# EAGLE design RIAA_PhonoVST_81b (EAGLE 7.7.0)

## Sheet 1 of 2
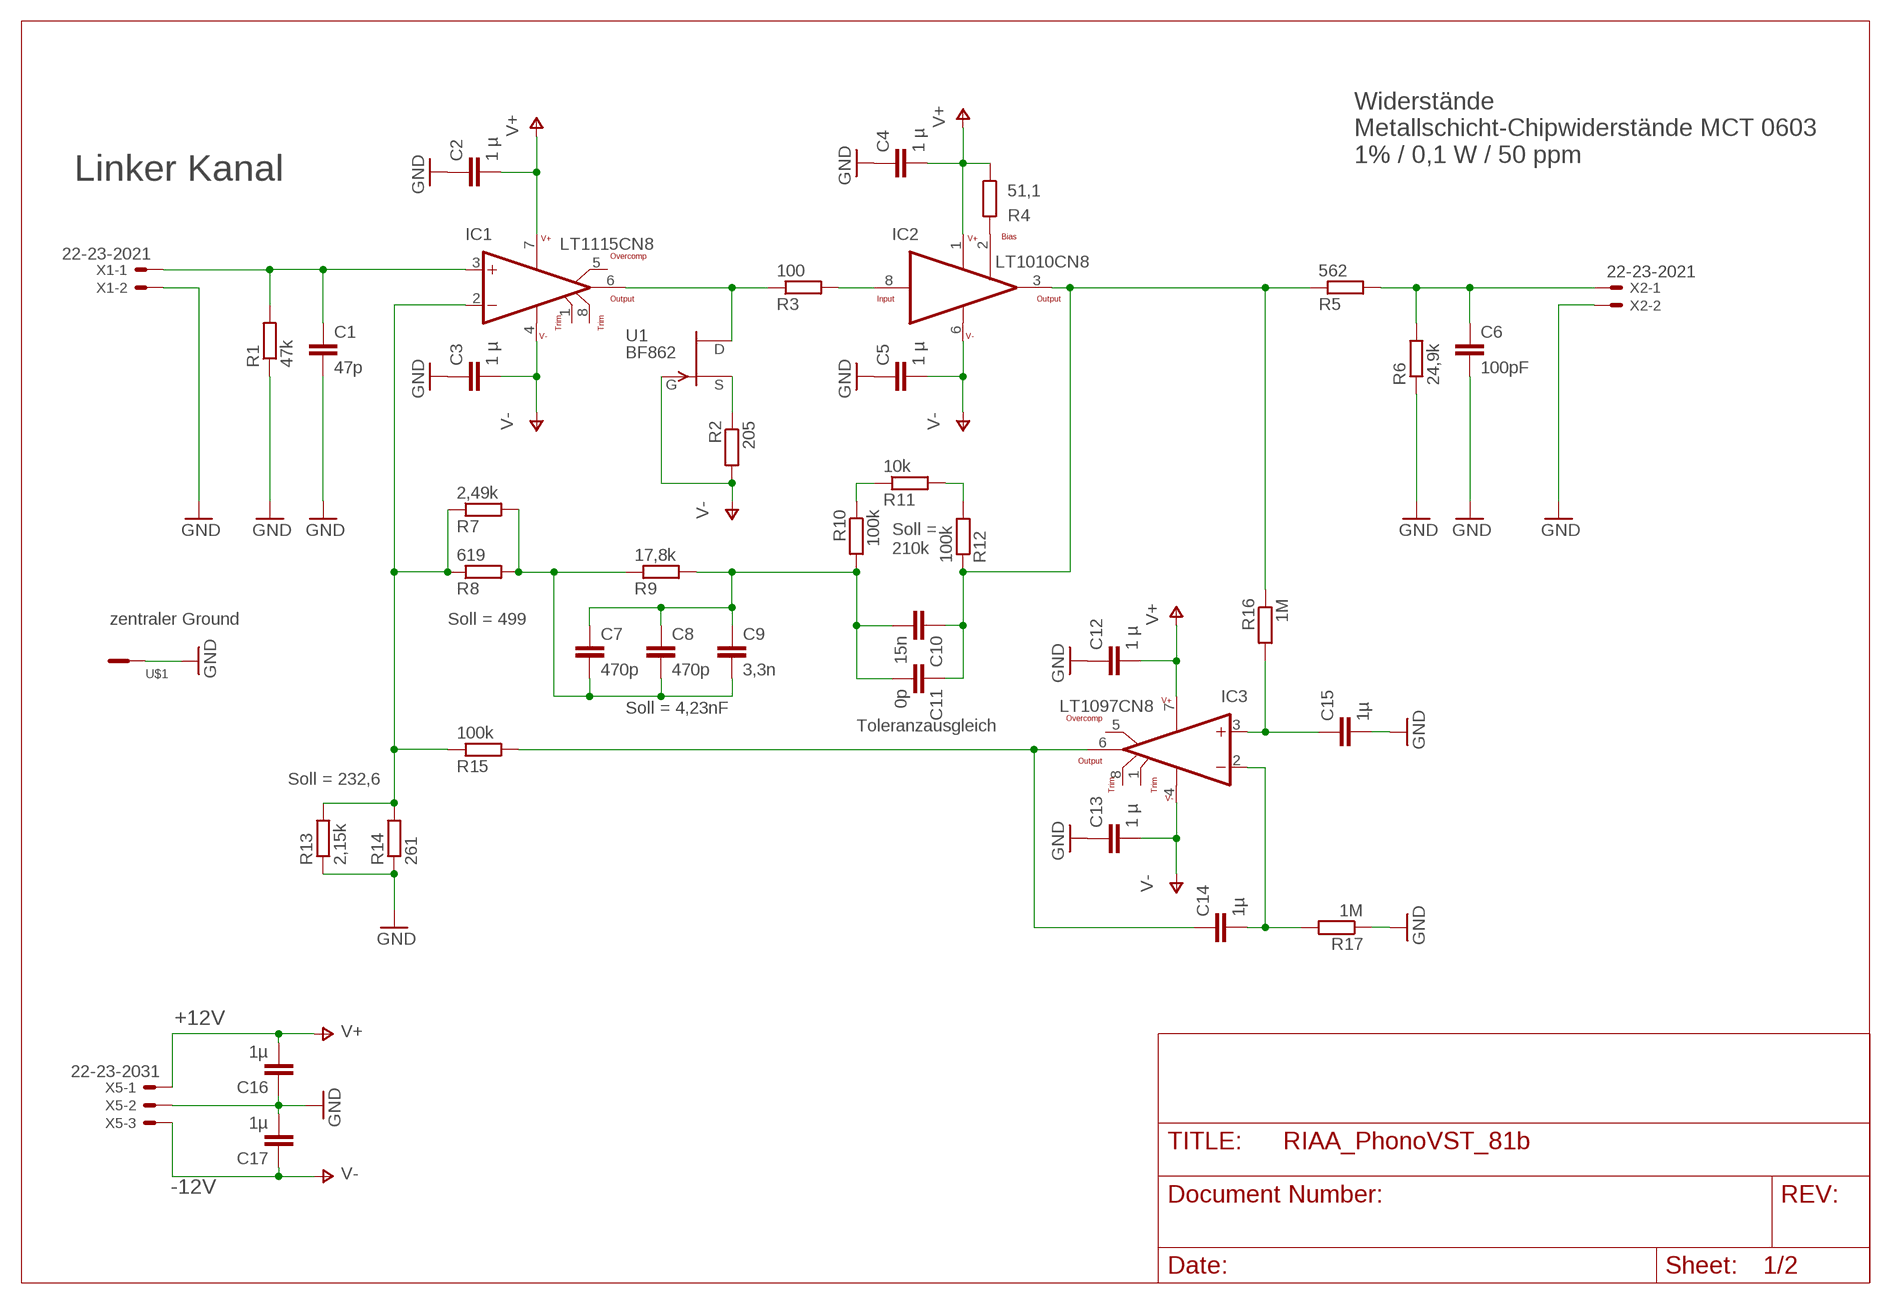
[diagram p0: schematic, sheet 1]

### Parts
C1  47p  C-EUC0603  [C0603]
C2  1 µ  C-EUC1206  [C1206]
C3  1 µ  C-EUC1206  [C1206]
C4  1 µ  C-EUC1206  [C1206]
C5  1 µ  C-EUC1206  [C1206]
C6  100pF  C-EUC0805  [C0805]
C7  470p  C-EUC2012  [C2012]
C8  470p  C-EUC2012  [C2012]
C9  3,3n  C-EUC3225  [C3225]
C10  15n  C-EUC3225  [C3225]
C11  0p  C-EUC2012  [C2012]
C12  1 µ  C-EUC1206  [C1206]
C13  1 µ  C-EUC1206  [C1206]
C14  1µ  C-EUC1206  [C1206]
C15  1µ  C-EUC1206  [C1206]
C16  1µ  C-EUC1206  [C1206]
C17  1µ  C-EUC1206  [C1206]
IC1  LT1115CN8  [DIL08]
IC2  LT1010CN8  [DIL08]
IC3  LT1097CN8  [DIL08]
R1  47k  R-EU_R0603  [R0603]
R2  205  R-EU_R0603  [R0603]
R3  100  R-EU_R0603  [R0603]
R4  51,1  R-EU_R0603  [R0603]
R5  562  R-EU_R0603  [R0603]
R6  24,9k  R-EU_R0603  [R0603]
R7  2,49k  R-EU_R0603  [R0603]
R8  619  R-EU_R0603  [R0603]
R9  17,8k  R-EU_R0603  [R0603]
R10  100k  R-EU_R0603  [R0603]
R11  10k  R-EU_R0603  [R0603]
R12  100k  R-EU_R0603  [R0603]
R13  2,15k  R-EU_R0603  [R0603]
R14  261  R-EU_R0603  [R0603]
R15  100k  R-EU_R0603  [R0603]
R16  1M  R-EU_R0603  [R0603]
R17  1M  R-EU_R0603  [R0603]
U1  BF862  [SOT23]
U$1  2FEET  [2FEETS]
X1  22-23-2021  [22-23-2021]
X2  22-23-2021  [22-23-2021]
X5  22-23-2031  [22-23-2031]

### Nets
GND: C1.2 C2.1 C3.1 C4.1 C5.1 C6.2 C12.1 C13.1 C15.2 C16.1 C17.2 R1.1 R6.1 R13.1 R14.1 R17.1 U$1.P$1 X1.2 X2.2 X5.2 ; also sheet 2
IC1: C1.1 IC1.3(+IN) R1.2 X1.1
IC2: IC2.8(INPUT) R3.2
IC3: C15.1 IC3.3(+IN) R16.2
N$1: C14.1 IC3.6(OUTPUT) R15.2
N$2: R2.1 U1.1(S)
N$3: IC2.2(BIAS) R4.2
N$5: C6.1 R5.2 R6.2 X2.1
N$7: C7.2 C8.2 C9.2 R7.2 R8.2 R9.1
N$8: C7.1 C8.1 C9.1 C10.2 C11.2 R9.2 R10.2
N$9: C14.2 IC3.2(-IN) R17.2
N$10: IC1.6(OUTPUT) R3.1 U1.2(D)
N$11: C10.1 C11.1 IC2.3(OUTPUT) R5.1 R12.1 R16.1
N$12: IC1.2(-IN) R7.1 R8.1 R13.2 R14.2 R15.1
N$13: R10.1 R11.1
N$17: R11.2 R12.2
V+: C2.2 C4.2 C12.2 C16.2 IC1.7(V+) IC2.1(V+) IC3.7(V+) R4.1 X5.1 ; also sheet 2
V-: C3.2 C5.2 C13.2 C17.1 IC1.4(V-) IC2.6(V-) IC3.4(V-) R2.2 U1.3(G) X5.3 ; also sheet 2
Unconnected: IC1.1(TRIM1) IC1.5(OVERCOMP) IC1.8(TRIM2) IC3.1(TRIM1) IC3.5(OVERCOMP) IC3.8(TRIM2)

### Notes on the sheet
- Widerstände
  Metallschicht-Chipwiderstände MCT 0603
  1% / 0,1 W / 50 ppm
- Linker Kanal
- Soll =
  210k
- zentraler Ground | Soll = 499
- Soll = 4,23nF
- Toleranzausgleich
- Soll = 232,6
- +12V
- -12V

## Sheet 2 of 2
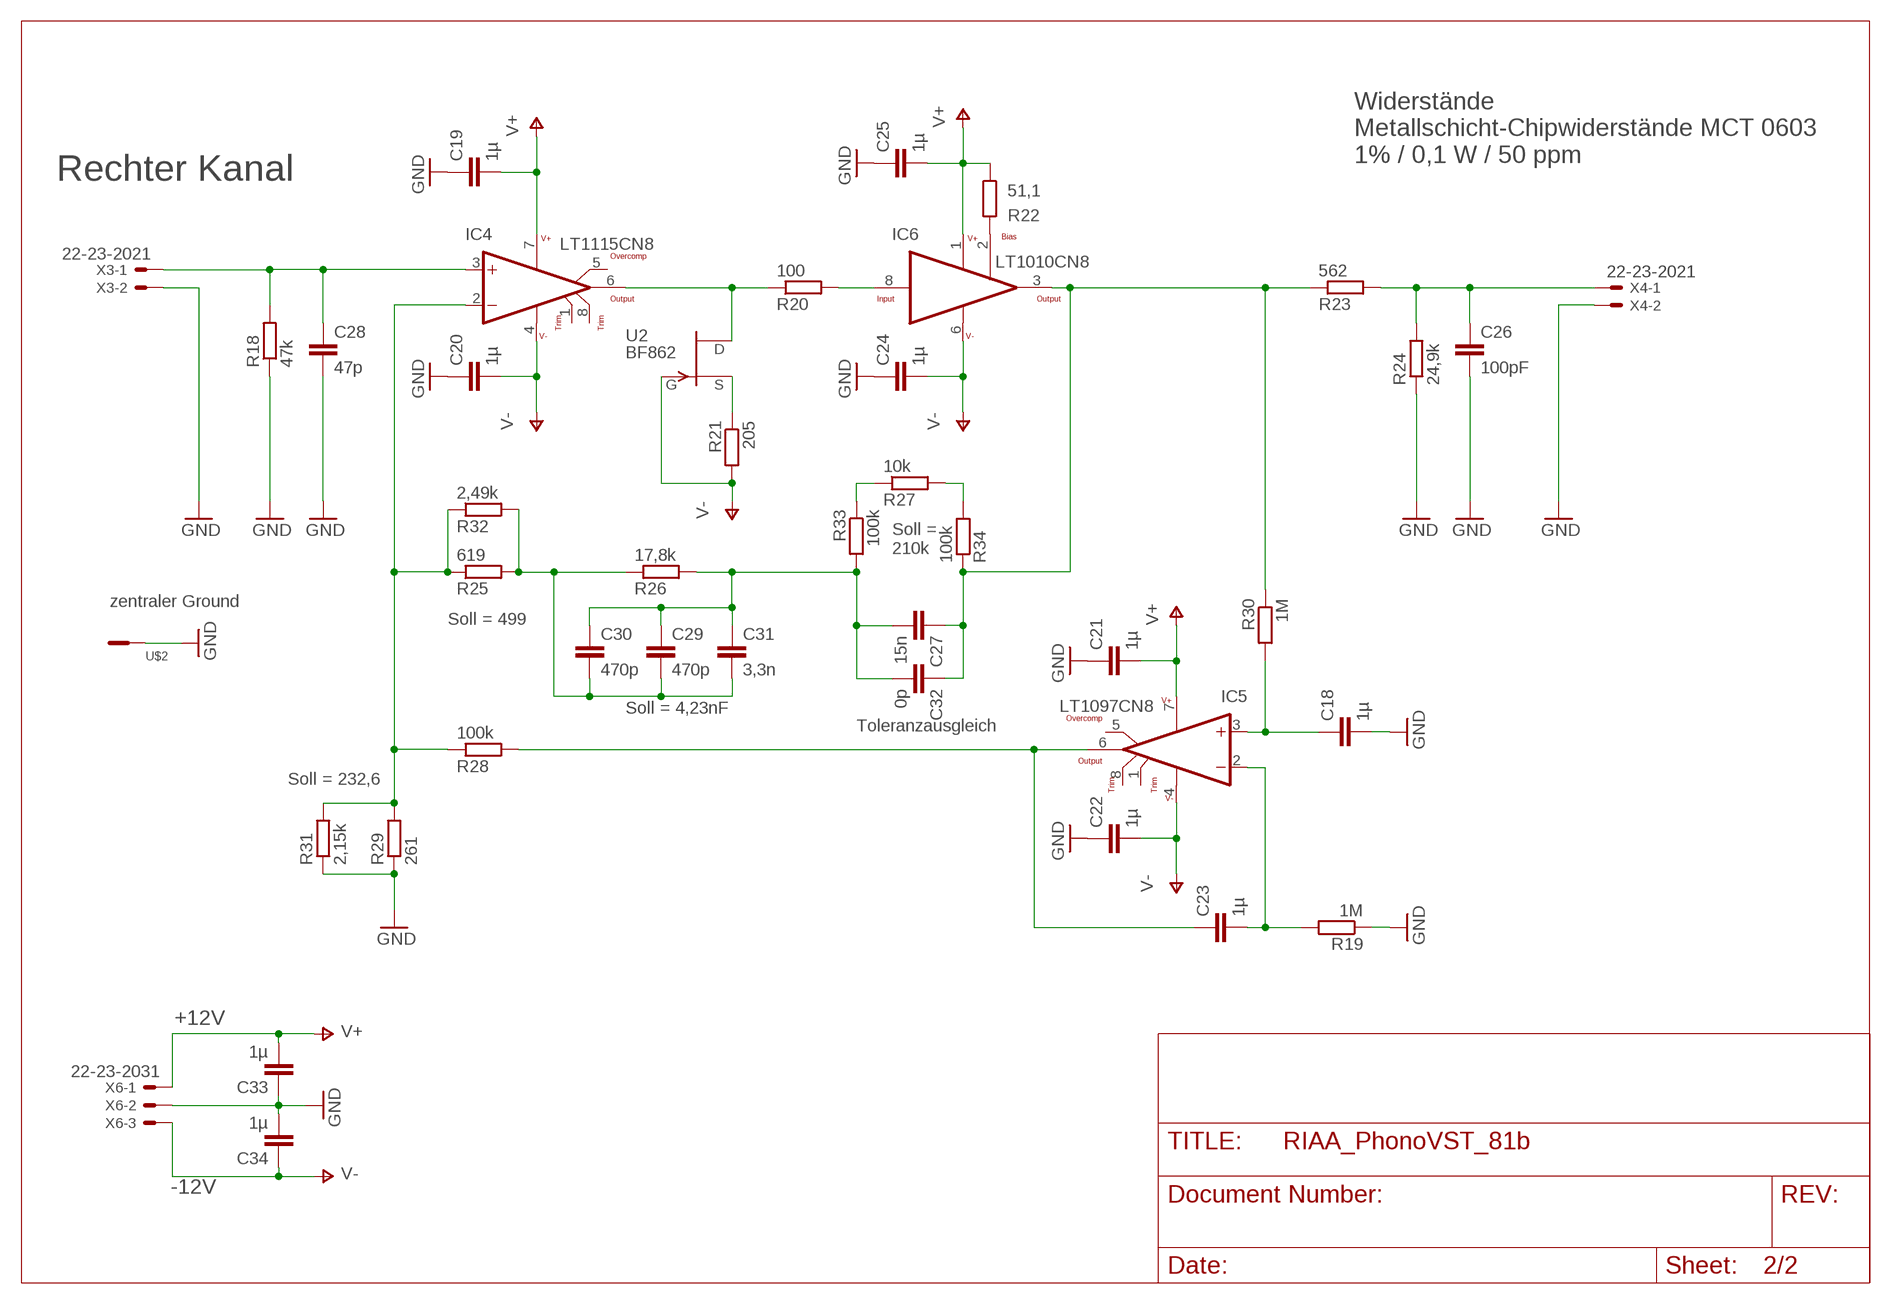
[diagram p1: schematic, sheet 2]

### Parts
C18  1µ  C-EUC1206  [C1206]
C19  1µ  C-EUC1206  [C1206]
C20  1µ  C-EUC1206  [C1206]
C21  1µ  C-EUC1206  [C1206]
C22  1µ  C-EUC1206  [C1206]
C23  1µ  C-EUC1206  [C1206]
C24  1µ  C-EUC1206  [C1206]
C25  1µ  C-EUC1206  [C1206]
C26  100pF  C-EUC0805  [C0805]
C27  15n  C-EUC3225  [C3225]
C28  47p  C-EUC0603  [C0603]
C29  470p  C-EUC2012  [C2012]
C30  470p  C-EUC2012  [C2012]
C31  3,3n  C-EUC3225  [C3225]
C32  0p  C-EUC2012  [C2012]
C33  1µ  C-EUC1206  [C1206]
C34  1µ  C-EUC1206  [C1206]
IC4  LT1115CN8  [DIL08]
IC5  LT1097CN8  [DIL08]
IC6  LT1010CN8  [DIL08]
R18  47k  R-EU_R0603  [R0603]
R19  1M  R-EU_R0603  [R0603]
R20  100  R-EU_R0603  [R0603]
R21  205  R-EU_R0603  [R0603]
R22  51,1  R-EU_R0603  [R0603]
R23  562  R-EU_R0603  [R0603]
R24  24,9k  R-EU_R0603  [R0603]
R25  619  R-EU_R0603  [R0603]
R26  17,8k  R-EU_R0603  [R0603]
R27  10k  R-EU_R0603  [R0603]
R28  100k  R-EU_R0603  [R0603]
R29  261  R-EU_R0603  [R0603]
R30  1M  R-EU_R0603  [R0603]
R31  2,15k  R-EU_R0603  [R0603]
R32  2,49k  R-EU_R0603  [R0603]
R33  100k  R-EU_R0603  [R0603]
R34  100k  R-EU_R0603  [R0603]
U2  BF862  [SOT23]
U$2  2FEET  [2FEETS]
X3  22-23-2021  [22-23-2021]
X4  22-23-2021  [22-23-2021]
X6  22-23-2031  [22-23-2031]

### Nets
GND: C18.2 C19.1 C20.1 C21.1 C22.1 C24.1 C25.1 C26.2 C28.2 C33.1 C34.2 R18.1 R19.1 R24.1 R29.1 R31.1 U$2.P$1 X3.2 X4.2 X6.2 ; also sheet 1
IC4: C28.1 IC4.3(+IN) R18.2 X3.1
IC5: IC6.8(INPUT) R20.2
IC6: C18.1 IC5.3(+IN) R30.2
N$18: C23.2 IC5.2(-IN) R19.2
N$19: IC4.6(OUTPUT) R20.1 U2.2(D)
N$20: C27.1 C32.1 IC6.3(OUTPUT) R23.1 R30.1 R34.1
N$21: C23.1 IC5.6(OUTPUT) R28.2
N$22: R21.1 U2.1(S)
N$23: IC6.2(BIAS) R22.2
N$24: C26.1 R23.2 R24.2 X4.1
N$25: C29.2 C30.2 C31.2 R25.2 R26.1 R32.2
N$26: C27.2 C29.1 C30.1 C31.1 C32.2 R26.2 R33.2
N$27: IC4.2(-IN) R25.1 R28.1 R29.2 R31.2 R32.1
N$28: R27.1 R33.1
N$29: R27.2 R34.2
V+: C19.2 C21.2 C25.2 C33.2 IC4.7(V+) IC5.7(V+) IC6.1(V+) R22.1 X6.1 ; also sheet 1
V-: C20.2 C22.2 C24.2 C34.1 IC4.4(V-) IC5.4(V-) IC6.6(V-) R21.2 U2.3(G) X6.3 ; also sheet 1
Unconnected: IC4.1(TRIM1) IC4.5(OVERCOMP) IC4.8(TRIM2) IC5.1(TRIM1) IC5.5(OVERCOMP) IC5.8(TRIM2)

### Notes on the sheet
- Widerstände
  Metallschicht-Chipwiderstände MCT 0603
  1% / 0,1 W / 50 ppm
- Rechter Kanal
- Soll =
  210k
- zentraler Ground
- Soll = 499
- Soll = 4,23nF
- Toleranzausgleich
- Soll = 232,6
- +12V
- -12V

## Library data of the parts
C1-C34 = rcl:C-EU: CAPACITOR, European symbol
IC1 IC4 = linear-technology:LT1115: Ultra-Low Noise, Low Distortion, Audio Op Amp
IC2 IC6 = linear-technology:LT1010: Fast ±150mA Power Buffer, Very Low Distortion Operation, 20MHz Bandwidth
IC3 IC5 = linear-technology:LT1097: Low Cost, Low Power Precision Op Amp
R1-R34 = rcl:R-EU_: RESISTOR, European symbol
U1 U2 = transistor-fet:BF862: N-channel junction FET
U$1 U$2 = Steckzungen:2FEET: Steckzunge Steckbreite: 2.8 mm Steckdicke: 0.8 mm 180 ° Unisoliert Metall Vogt Verbindungstechnik 3785q08.68
X1-X4 = con-molex:22-23-2021: .100" (2.54mm) Center Header - 2 Pin; MF: MOLEX; MPN: 22-23-2021; OC_FARNELL: 1462926; OC_NEWARK: 25C3832
X5 X6 = con-molex:22-23-2031: .100" (2.54mm) Center Header - 3 Pin; MF: MOLEX; MPN: 22-23-2031; OC_FARNELL: 1462950; OC_NEWARK: 30C0862

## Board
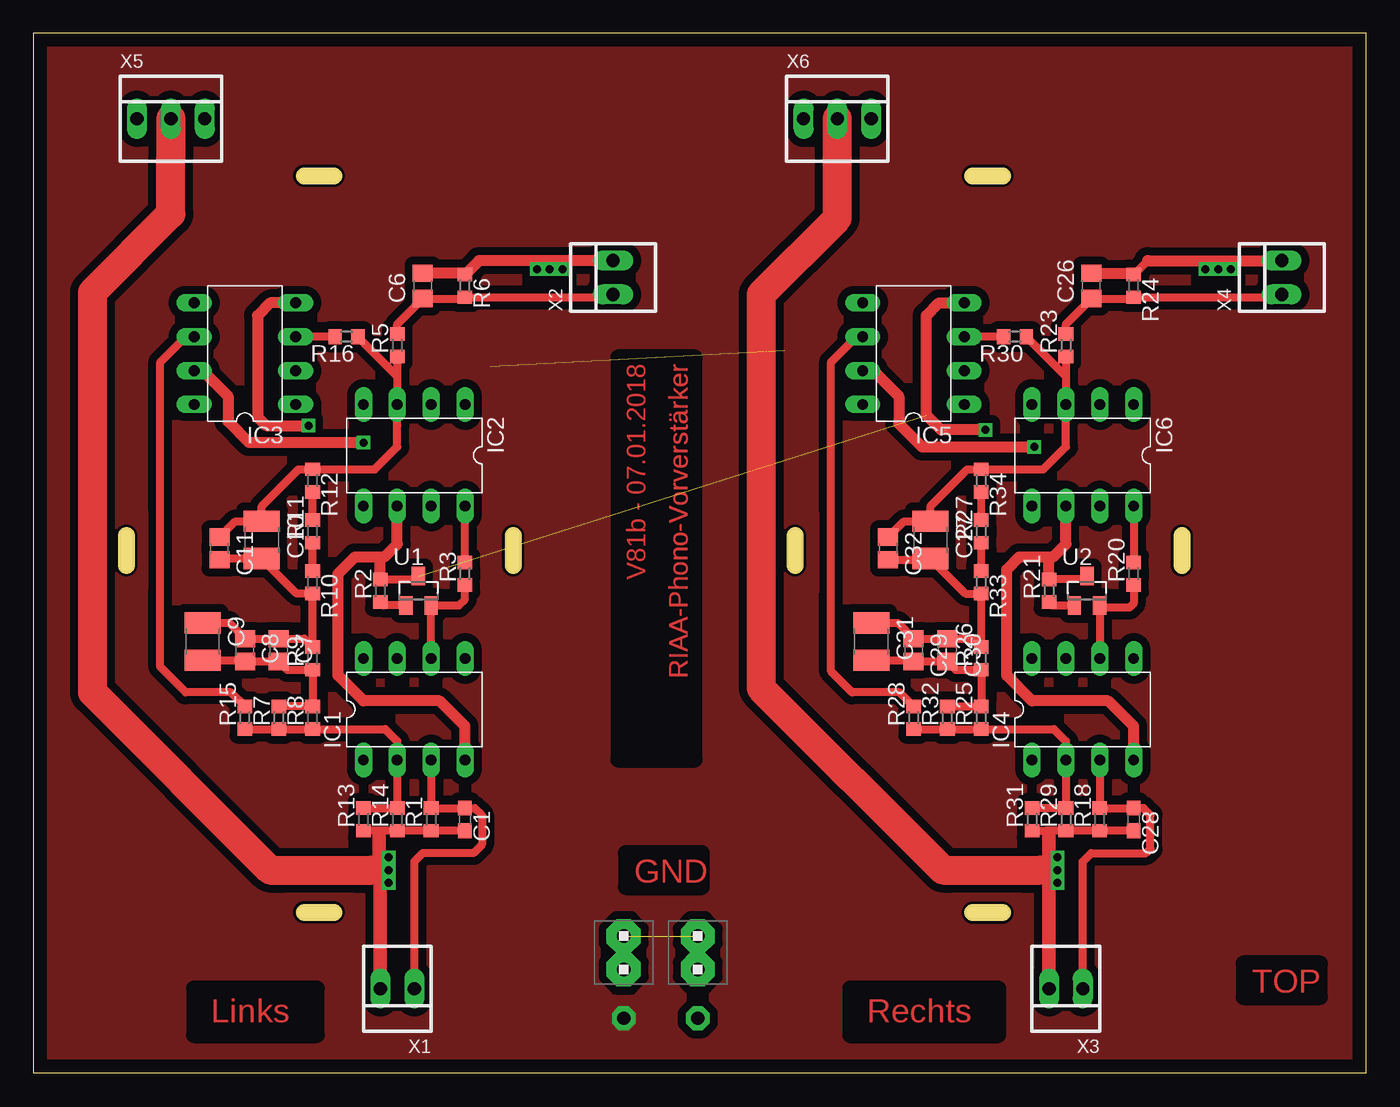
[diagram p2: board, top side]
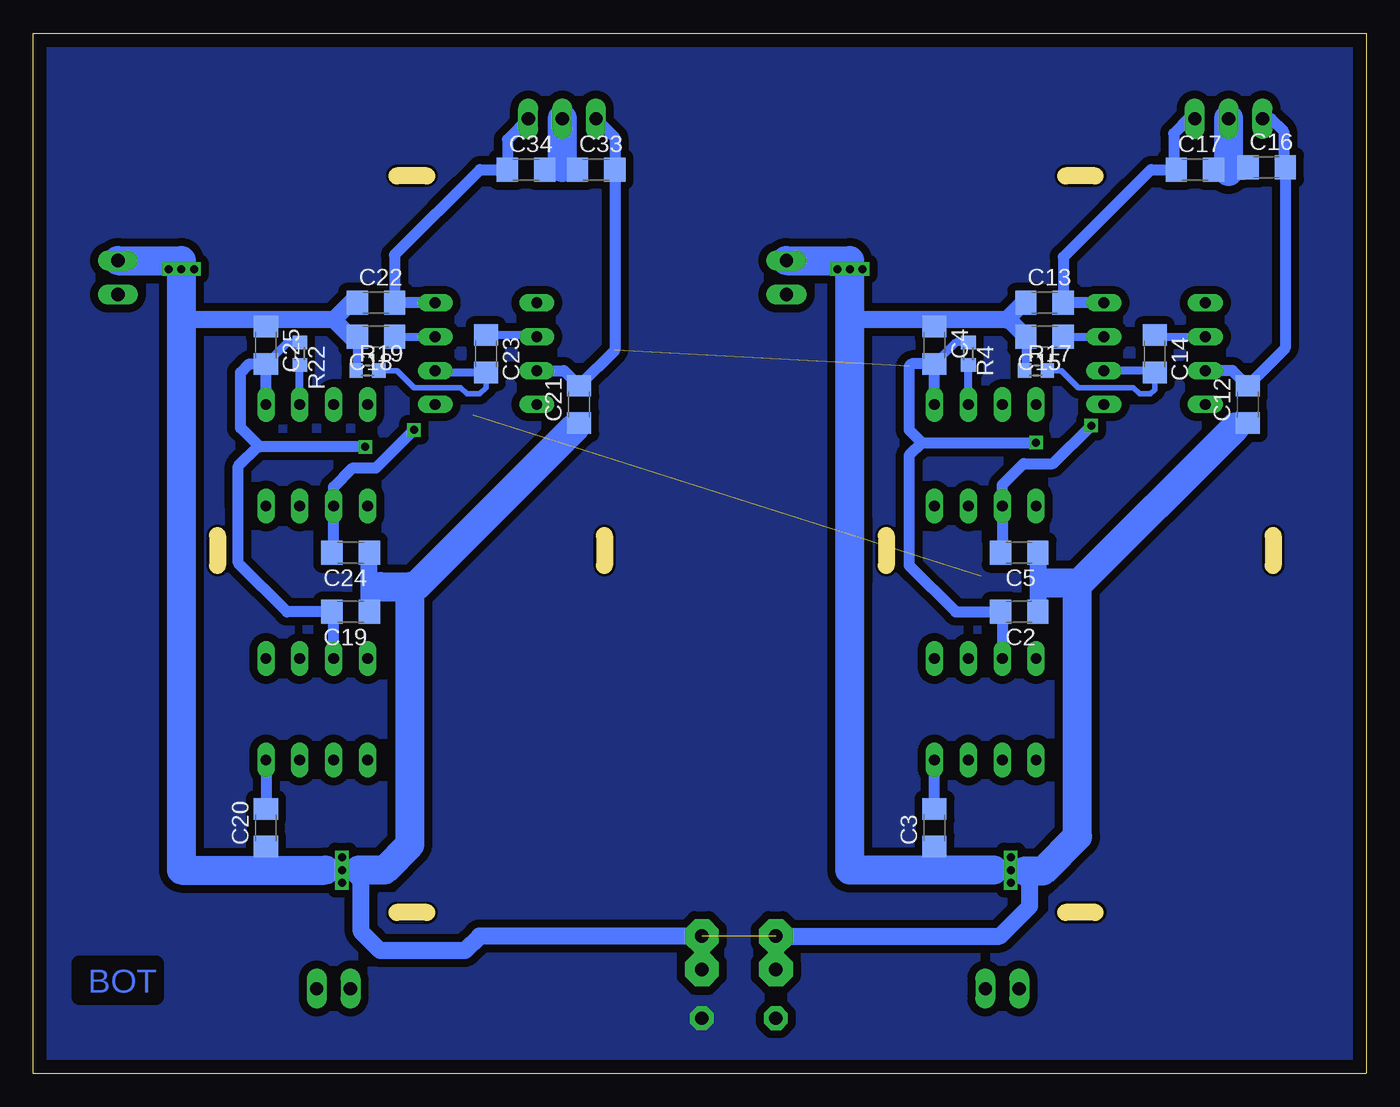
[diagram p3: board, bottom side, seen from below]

Size 100 x 78 mm. Coordinates in mm from the lower left corner, seen from the top.
Outline: 100,0 100,78 0,78 0,0 100,0
Copper layers (1*16): Top 0.035mm / dielectric 1.5mm / Bottom 0.035mm
Design rules "default": minimum track width 10mil, minimum drill 24mil, track to track 8mil, track to pad 8mil, pad to pad 8mil, via to via 8mil, smd to smd 8mil, copper to edge 40mil, drill to drill 8mil, minimum pad ring 10mil, minimum via ring 8mil, stop-mask expansion 4mil, vias tented up to drill 0mil, thermal gap 10mil
tRestrict: area 12.1,2.9 to 21.3,6.3; area 61.3,2.9 to 72.4,6.3; area 44.5,14 to 50.2,16.5; area 90.8,5.7 to 96.5,8.3; area 43.9,23.5 to 49.6,53.7; 8 lines
bRestrict: area 90.8,5.7 to 96.5,8.3; 8 lines
Milling: 8 lines

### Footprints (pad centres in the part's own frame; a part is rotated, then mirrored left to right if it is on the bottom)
C0603 = smd 1.1 x 1: 1 -0.85,0; 2 0.85,0
C1206 = smd 1.6 x 1.8: 1 -1.4,0; 2 1.4,0
C0805 = smd 1.3 x 1.5: 1 -0.95,0; 2 0.95,0
C2012 = smd 1.3 x 1.5: 1 -0.85,0; 2 0.85,0
C3225 = smd 1.6 x 2.7: 1 -1.4,0; 2 1.4,0
DIL08 = drill 0.813 long: 1 -3.81,-3.81; 2 -1.27,-3.81; 3 1.27,-3.81; 4 3.81,-3.81; 5 3.81,3.81; 6 1.27,3.81; 7 -1.27,3.81; 8 -3.81,3.81
R0603 = smd 1 x 1.1: 1 -0.85,0; 2 0.85,0
SOT23 = smd 1 x 1.4: 1 -0.95,-1.1; 2 0.95,-1.1; 3 0,1.1
2FEETS = drill 1 pad 2.54 octagon: P$1 -1.25,0; P$2 1.25,0
22-23-2021 = drill 1 long: 1 -1.27,0; 2 1.27,0
22-23-2031 = drill 1 long: 1 -2.54,0; 2 0,0; 3 2.54,0

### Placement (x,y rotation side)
C1  32.38,19.05 270 top
C2  26.04,34.61 180 bottom
C3  32.38,18.41 90 bottom
C4  32.38,54.61 270 bottom
C5  26.04,39.05 180 bottom
C6  29.21,59.05 90 top
C7  18.41,31.75 270 top
C8  15.88,31.75 270 top
C9  12.7,32.38 270 top
C10  17.14,40.01 270 top
C11  13.97,39.37 270 top
C12  8.89,50.16 90 bottom
C13  24.13,57.78 0 bottom
C14  15.88,53.98 270 bottom
C15  24.13,55.24 180 bottom
C16  7.47,67.94 0 bottom
C17  12.85,67.79 0 bottom
C18  74.3,55.24 180 bottom
C19  76.2,34.61 180 bottom
C20  82.55,18.41 90 bottom
C21  59.05,50.16 90 bottom
C22  74.3,57.78 0 bottom
C23  66.04,53.98 270 bottom
C24  76.2,39.05 180 bottom
C25  82.55,54.61 270 bottom
C26  79.38,59.05 90 top
C27  67.31,40.01 270 top
C28  82.55,19.05 270 top
C29  66.04,31.75 270 top
C30  68.58,31.75 270 top
C31  62.87,32.38 270 top
C32  64.14,39.37 270 top
C33  57.77,67.79 0 bottom
C34  63.03,67.79 0 bottom
IC1  28.57,27.3 0 top
IC2  28.57,46.35 180 top
IC3  15.88,53.98 90 top
IC4  78.74,27.3 0 top
IC5  66.04,53.98 90 top
IC6  78.74,46.35 180 top
R1  29.84,19.05 90 top
R2  26.04,36.2 90 top
R3  32.38,37.47 90 top
R4  29.84,53.98 270 bottom
R5  27.3,54.61 90 top
R6  32.38,59.05 270 top
R7  18.41,26.67 90 top
R8  20.95,26.67 90 top
R9  20.95,31.11 90 top
R10  20.95,36.83 270 top
R11  20.95,40.64 90 top
R12  20.95,44.45 270 top
R13  24.77,19.05 90 top
R14  27.3,19.05 90 top
R15  15.88,26.67 90 top
R16  23.5,55.24 180 top
R17  24.77,52.7 0 bottom
R18  80.01,19.05 90 top
R19  74.93,52.7 0 bottom
R20  82.55,37.47 90 top
R21  76.2,36.2 90 top
R22  80.01,53.98 270 bottom
R23  77.47,54.61 90 top
R24  82.55,59.05 270 top
R25  71.12,26.67 90 top
R26  71.12,31.11 90 top
R27  71.12,40.64 90 top
R28  66.04,26.67 90 top
R29  77.47,19.05 90 top
R30  73.66,55.24 180 top
R31  74.93,19.05 90 top
R32  68.58,26.67 90 top
R33  71.12,36.83 270 top
R34  71.12,44.45 270 top
U1  28.89,36.2 0 top
U2  79.06,36.2 0 top
U$1  44.29,9.05 270 top
U$2  49.85,9.05 270 top
X1  27.3,6.35 180 top
X2  43.5,59.69 90 top
X3  77.47,6.35 180 top
X4  93.66,59.69 90 top
X5  10.32,71.6 0 top
X6  60.33,71.6 0 top

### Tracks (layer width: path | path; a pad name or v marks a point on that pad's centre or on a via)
GND  (via drill 0.6)  (1 unrouted)
  Top 0.254: 25.95,17.91 26.05,18.19 R14.1 27.28,18.22 27.23,18.21
  Top 0.305: 25.4,15.24 26.11,15.24 v26.67,15.24 | v38.73,60.33 38.73,60.96
  Top 0.61: 27.23,18.21 R13.1 | 25.94,15.72 26.11,15.72 26.11,15.24 | 82.45,60.01 R24.1 83.61,60.96 | 75.56,15.24 76.2,15.24 v76.83,15.24 | C28.2 R18.1 R29.1 76.22,18.2 76.2,18.02 76.02,18.2 R31.1 | R1.1 C1.2 R14.1
  Top 0.813: C6.2 32.28,60.01 R6.1 33.44,60.96 38.73,60.96 X2.2 | 25.94,15.72 25.88,15.72 25.8,15.72 25.8,15.82 | 10.32,68.89 10.32,68.71 | C26.2 82.45,60.01 | 83.61,60.96 X4.2
  Top 1.016: 25.95,17.91 25.94,15.72 | X3.2 76.2,15.24 76.2,18.02 | X1.2 26.04,15.57 25.88,15.72
  Top 2.184: X5.2 10.32,68.71 10.32,64.45 4.45,58.58 4.45,28.57 17.78,15.24 25.4,15.24 | 75.56,15.24 68.26,15.24 54.61,28.89 54.61,58.42 60.33,64.14 X6.2
  Bottom 0.254: R17.1 25.53,52.79
  Bottom 0.305: 27.94,15.24 v26.67,15.24 | C3.1 32.38,15.24 | 59.37,48.42 59.05,48.74 C21.1
  Bottom 0.406: 25.88,14.92 25.88,15.24 | 76.04,15.08 76.68,15.08 v76.83,15.24
  Bottom 0.61: 25.53,52.79 C15.2 | 9.8,48.47 9.51,48.77 C12.1 | R19.1 75.69,52.79 C18.2 | C19.1 74.8,35.69 73.98,36.51 | 75.56,15.24 v76.83,15.24 78.11,15.24 | C25.1 82.87,56.33 82.87,56.52 | C20.1 82.55,15.4 82.39,15.24 | C33.1 59.17,67.94 60.33,67.94 61.63,67.94 C34.2
  Bottom 0.813: 24.11,36.77 24.64,37.2 24.64,37.27 | 38.73,60.96 v38.73,60.33
  Bottom 1.27: U$1.P$1 27.48,10.3 25.24,12.54 25.24,14.29 25.88,14.92 | U$2.P$1 66.54,10.3 67.63,9.21 73.98,9.21 75.41,10.64 75.41,14.45 76.04,15.08 | C5.1 24.64,37.27 C2.1 | C15.2 26.8,56.52 26.99,56.52 | 26.99,56.52 31.88,56.52 | 31.88,56.52 C4.1 | 31.88,56.52 38.73,56.52 | C13.1 25.72,57.78 26.99,56.52 | 25.61,15.17 25.68,15.24 25.88,15.24 v26.67,15.24 | C19.1 C24.1 | 88.77,56.01 88.9,55.88 | C22.1 76.2,57.78 77.47,56.52 | C18.2 76.2,55.24 77.47,56.52 | 77.47,56.52 82.87,56.52 88.9,56.52 | C16.1 9.19,67.63 10.32,67.63 | C17.2 10.32,67.79
  Bottom 2.184: 27.94,15.24 32.38,15.24 38.73,15.24 38.73,56.52 v38.73,60.33 | 21.66,36.63 21.66,17.78 24.27,15.17 25.61,15.17 | 21.66,36.63 21.82,36.77 24.11,36.77 | 21.66,36.63 9.82,48.47 9.8,48.47 | X2.2 38.73,60.96 | 71.75,36.51 71.31,36.51 59.4,48.42 59.37,48.42 | 73.98,36.51 71.75,36.51 | 71.75,36.51 71.75,17.14 73.66,15.24 75.56,15.24 | X4.2 88.9,60.96 v88.9,60.33 88.9,56.52 88.9,55.88 88.9,15.24 82.39,15.24 78.11,15.24 | X6.2 60.33,67.94 | 10.32,67.63 10.32,67.79 X5.2
IC1
  Top 0.61: IC1.3 R1.2 C1.1 33.13,19.9 33.66,19.38 33.66,17.14 33.02,16.51 29.21,16.51 28.57,15.88 X1.1
IC2
  Top 0.61: R3.2 IC2.8
IC3
  Top 0.61: R16.2 IC3.3
  Bottom 0.61: C15.1 IC3.3
IC4
  Top 0.61: X3.1 78.74,15.88 79.38,16.51 83.5,16.51 83.82,16.83 83.82,19.37 83.29,19.9 C28.1 R18.2 IC4.3
IC5
  Top 0.61: IC6.8 R20.2
IC6
  Top 0.61: R30.2 IC5.3
  Bottom 0.61: C18.1 IC5.3
N$1
  Top 0.61: R15.2 14.82,28.57 11.43,28.57 9.53,30.48 9.53,53.34 11.43,55.24 IC3.6
  Bottom 0.406: C14.1 15.74,55.24
  Bottom 0.61: 15.74,55.24 IC3.6
N$2
  Top 0.61: U1.1 26.29,35.09 R2.1
N$3
  Bottom 0.61: IC2.2 R4.2
N$4  (via drill 0.6)
  other vias: 26.67,16.19
N$5
  Top 0.406: 32.28,58.1 R6.2 | 43.28,58.2 X2.1
  Top 0.61: R5.2 27.3,56.2 C6.1 32.28,58.1 | R6.2 43.28,58.2
N$6  (via drill 0.6)
  other vias: 26.67,14.29
N$7
  Top 0.254: 15.79,30.98 C8.2
  Top 0.61: C9.2 15.79,30.98 | C8.2 C7.2 19.05,30.27 R9.1 R8.2 R7.2
N$8
  Top 0.305: 14.05,38.6 C11.2
  Top 0.61: C9.1 14.69,33.78 C8.1 C7.1 20.32,32.6 R9.2 R10.2 19.77,35.98 C10.2 14.05,38.6
N$9
  Bottom 0.406: 16,52.7 C14.2 15.88,51.28 16.19,50.96 16.99,50.96 17.46,51.44 21.59,51.44 22.86,52.7 R17.2 | 19.05,52.7 IC3.2
  Bottom 0.61: 16,52.7 19.05,52.7
N$10
  Top 0.305: IC1.6 29.84,31.43
  Top 0.61: 29.84,31.43 U1.2 31.92,35.09 32.38,35.56 R3.1
N$11
  Top 0.254: 27.3,52.28 IC2.3
  Top 0.305: 27.3,48.26 27.3,48.58
  Top 0.61: R16.1 27.3,52.28 | C11.1 15.15,41.41 C10.1 17.14,42.55 19.9,45.3 R12.1 25.61,45.3 27.3,46.99 27.3,48.58 IC2.3 R5.1
N$12
  Top 0.61: R13.2 R14.2 IC1.2 27.3,24.92 26.41,25.82 R8.1 R7.1 R15.1
N$13
  Top 0.61: R10.1 R11.1
N$14  (via drill 0.6)
  other vias: 37.78,60.33
N$15  (via drill 0.6)
  other vias: 39.69,60.33
N$17
  Top 0.61: R11.2 R12.2
N$18
  Bottom 0.406: R19.2 72.71,52.7 71.44,51.44 67.94,51.44 67.47,50.96 66.52,50.96 66.04,51.44 C23.2
  Bottom 0.61: IC5.2 69.72,52.58 C23.2
N$19
  Top 0.61: R20.1 82.55,35.24 82.23,34.92 80.18,34.92 U2.2 IC4.6
N$20
  Top 0.61: C32.1 65.32,41.41 C27.1 67.31,42.55 70.06,45.3 R34.1 75.78,45.3 77.47,46.99 IC6.3 77.47,52.39 | R23.1 77.47,52.39 | R30.1 77.37,52.39 77.47,52.39
N$21
  Top 0.61: R28.2 64.98,28.57 61.44,28.57 59.85,30.16 59.85,53.34 61.75,55.24 IC5.6
  Bottom 0.61: IC5.6 62.36,55.38 C23.1
N$22
  Top 0.61: R21.1 76.45,35.09 U2.1
N$23
  Bottom 0.61: IC6.2 R22.2
N$24
  Top 0.61: R23.2 77.47,56.2 C26.1 82.45,58.1 R24.2 93.45,58.2 X4.1
N$25
  Top 0.61: R32.2 R25.2 R26.1 69.22,30.27 C30.2 C29.2 65.95,30.98 C31.2
N$26
  Top 0.61: C31.1 64.86,33.78 C29.1 C30.1 70.48,32.6 R26.2 R33.2 69.94,35.98 C27.2 67.22,38.52 C32.2
N$27
  Top 0.61: R28.1 R32.1 R25.1 76.57,25.82 77.47,24.92 IC4.2 R29.2 R31.2 74.87,19.84
N$28
  Top 0.61: R33.1 R27.1
N$29
  Top 0.61: R27.2 R34.2
N$30  (via drill 0.6)
  other vias: 76.83,16.19
N$31  (via drill 0.6)
  other vias: 76.83,14.29
N$32  (via drill 0.6)
  other vias: 89.85,60.33
N$33  (via drill 0.6)
  other vias: 87.95,60.33
N$34  (via drill 1 pad 1.78)
  other vias: 49.85,4.13
  pour Bottom (isolate 0.61): 48.26,2.54 51.44,2.54 51.44,5.71 48.26,5.71
N$35  (via drill 1 pad 1.78)
  other vias: 44.29,4.13
  pour Top (isolate 0.61): 42.7,2.54 45.88,2.54 45.88,5.71 42.7,5.71
N$37
  pour Top (isolate 0.6): 0,78 0,0 100,0 100,78
  pour Bottom (isolate 0.6): 0,78 0,0 99.9,0 99.9,78
  pour Top: 56.44,42.07 58.82,42.03 58.82,36.08 56.44,36.12
  pour Top: 84.73,37.82 84.73,41.83 84.81,41.83 87.63,41.83 87.63,36.95 87.63,36.71 85.37,36.71 84.73,36.71
  pour Top: 69.12,70.3 74.24,70.3 74.14,66.16 74.14,65.88 69.02,65.88 69.12,69.98
  pour Top (rank 3): 68.98,13.41 69.02,10.6 74.18,10.6 74.14,13.41
  pour Top: 34.57,40.56 34.57,41.79 37.27,41.79 37.43,41.79 37.43,36.91 37.43,36.67 34.81,36.67 34.57,36.67
  pour Top: 6.27,42.15 8.49,42.11 8.49,36.43 6.27,36.43
  pour Top: 19.95,68.83 23.97,68.78 23.97,65.88 18.89,65.88 18.89,68.78
  pour Top: 18.89,12.1 18.89,10.64 23.73,10.64 23.97,10.64 23.97,13.1 23.97,13.41 19.05,13.41 18.89,13.41
  pour Bottom (rank 2): 71.08,13.45 74.02,13.45 74.02,13.14 74.02,11.11 73.7,10.79 73.5,10.6 68.94,10.6 68.94,13.06 69.33,13.45
  pour Bottom: 56.83,41.75 58.58,41.75 58.58,37.23 58.58,36.67 56.2,36.67 55.72,36.67 55.72,41.47 55.72,41.75
  pour Bottom: 87.07,42.43 87.07,36.2 85.76,36.16 85.76,42.39
  pour Bottom: 84.45,36.43 84.45,36.51 84.77,36.83 85.8,37.86 85.8,36.43
  pour Bottom: 6.67,41.75 8.45,41.75 8.45,37.66 8.45,36.67 5.99,36.67 5.52,36.67 5.52,41.12 5.52,41.75
  pour Bottom: 22.54,65.05 20.45,65.11 18.1,67.45 18.1,67.47 19.41,68.78 23.22,68.78 24.01,67.98 24.01,66.52
  pour Bottom: 70.74,65.2 70.69,65.2 68.4,67.49 68.4,67.51 69.77,70.31 73.56,70.31 74.19,68.05 74.19,66.34 73.61,65.76 71.3,65.76
  pour Bottom: 34.67,36.65 34.67,36.88 35.38,37.59 35.38,36.83
  pour Bottom: 35.43,42.16 36.91,42.14 36.91,36.09 35.43,36.09
  pour Bottom (rank 2): 24.57,11.31 23.73,12.14 23.73,13.26 22.62,14.25 20.12,14.25 18.73,12.86 18.73,11.39 19.68,10.44 23.69,10.44
  pour Bottom (rank 2): 72.03,14.21 72.11,14.21 72.35,13.97 72.91,13.41 72.11,13.41 72.03,13.49
V+  (via drill 0.6)  (1 unrouted)
  Top 0.813: v24.77,47.31 16.19,47.31 14.61,48.9 14.61,50.8 12.7,52.7 IC3.7 | IC5.7 63.02,52.7 64.93,50.8 64.93,48.74 66.67,46.99 v75.09,46.99
  Bottom 0.406: C2.2 27.3,34.8
  Bottom 0.61: R4.1 30.77,54.83 C4.2 | C25.2 80.94,54.83 R22.1
  Bottom 0.813: IC2.1 C4.2 34.1,53.21 34.29,53.02 34.29,48.26 33.34,47.31 | 27.3,34.8 IC1.7 | IC3.7 10.03,52.7 C12.2 6.07,54.38 C16.2 6.19,67.83 6.19,70.64 7.14,71.6 X5.1 | 33.34,47.31 v24.77,47.31 | 33.34,47.31 34.29,46.35 34.29,38.1 30.8,34.61 C2.2 | IC6.1 C25.2 83.79,53.21 84.45,52.55 84.45,48.42 83.03,46.99 | IC5.7 60.2,52.7 C21.2 56.37,54.25 C33.2 56.37,70.19 X6.1 | IC4.7 77.47,34.48 C19.2 80.96,34.61 84.61,38.26 84.61,45.56 83.19,46.99 83.03,46.99 | v75.09,46.99 83.03,46.99
V-  (via drill 0.6)  (1 unrouted)
  Top 0.61: U2.3 78.81,37.05 R21.2 | 76.2,38.73 76.52,38.73 | R2.2 28.89,37.05 U1.3
  Top 0.813: IC3.4 17.78,57.78 16.83,56.83 16.83,49.21 17.46,48.58 v20.64,48.58 | IC1.4 32.38,26.04 30.48,27.94 24.77,27.94 22.86,29.84 22.86,37.47 24.13,38.73 26.04,38.73 | 26.04,38.73 26.35,38.73 27.3,39.69 IC2.6 | R2.2 26.04,38.73 | IC4.4 82.55,26.04 80.64,27.94 74.93,27.94 73.03,29.84 73.03,37.78 73.98,38.73 76.2,38.73 R21.2 | 76.52,38.73 77.47,39.69 IC6.6 | v71.44,48.26 68.1,48.26 66.99,49.37 66.99,56.83 67.94,57.78 IC5.4
  Bottom 0.813: C3.2 IC1.4 | IC3.4 C13.2 22.73,61.21 16.15,67.79 C17.1 14.45,67.67 14.45,70.48 13.34,71.6 X5.3 | v20.64,48.58 23.5,45.72 25.72,45.72 27.3,44.13 IC2.6 27.3,39.18 C5.2 | IC4.4 C20.2 | IC5.4 C22.2 72.89,61.39 66.5,67.79 C34.1 64.44,70.03 X6.3 | C24.2 77.47,39.18 IC6.6 77.47,43.97 76.04,45.4 74.3,45.4 v71.44,48.26

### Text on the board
Top: V81b - 07.01.2018 | RIAA-Phono-Vorverstärker | RIAA-Phono-Vorverstärker | GND | TOP | Links | Rechts
Bottom: BOT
